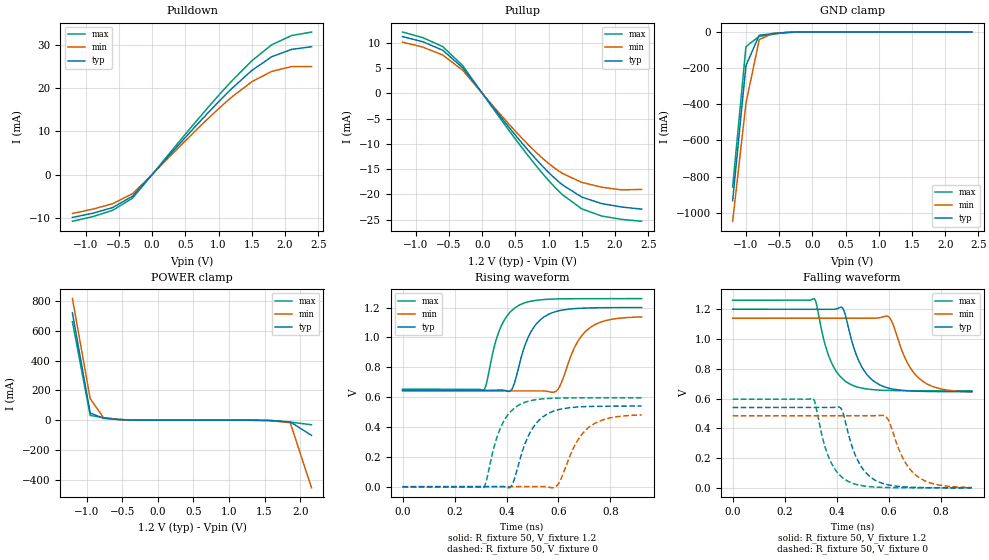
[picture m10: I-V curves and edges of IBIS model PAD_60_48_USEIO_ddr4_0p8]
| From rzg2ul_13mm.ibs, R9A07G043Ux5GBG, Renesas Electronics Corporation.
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[Model] PAD_60_48_USEIO_ddr4_0p8
Model_type I/O
Polarity   Non-Inverting
Vinl = 0.8670
Vinh = 1.0530
Vmeas= 0.960
| Capacitance   typ   min   max
C_comp   2.102e-12   2.013e-12   2.216e-12
[Model Spec]
| Subparameter   typ   min   max
Vmeas   0.960   0.912   1.008
Vinh   1.0530   1.0050   1.1010
Vinl   0.8670   0.8190   0.9150
| Variables   typ   min   max
[GND Clamp Reference]   0   0   0
[POWER Clamp Reference]   1.2   1.14   1.26
[Pulldown Reference]   0   0   0
[Pullup Reference]   1.2   1.14   1.26
[Temperature Range]   25   125   -40
[Voltage Range]   1.2   1.14   1.26
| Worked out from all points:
|   slope of the pulldown table from 0 to 0.18 V, typ, clamps not added: 57.7 ohm
|   slope of the pullup table from 0 to 0.18 V, typ, clamps not added: 59.2 ohm
|   GND clamp passes 1 mA (typ) near -0.30 V on its own axis
|   POWER clamp passes 1 mA (typ) near -0.38 V on its own axis
|   rising waveform, R_fixture 50, V_fixture 1.2: 20-80 % time 73.4ps typ, 82ps min, 66.5ps max; typ from 0.646 V to 1.2 V
|   rising waveform, R_fixture 50, V_fixture 0: 20-80 % time 78.4ps typ, 88.6ps min, 70.3ps max; typ from 0 V to 0.54 V
|   falling waveform, R_fixture 50, V_fixture 1.2: 20-80 % time 74.9ps typ, 84ps min, 68.9ps max; typ from 1.2 V to 0.646 V
|   falling waveform, R_fixture 50, V_fixture 0: 20-80 % time 73.8ps typ, 82.3ps min, 67.3ps max; typ from 0.54 V to 0 V
[GND Clamp]
| Voltage   I(typ)   I(min)   I(max)
-1.2V     -932.7mA   -1.047A    -857.4mA
-1V       -185.5mA   -394.3mA   -80.64mA
-800mV    -17.89mA   -41.9mA    -23.65mA
-600mV    -9.04mA    -7.411mA   -12.44mA
-400mV    -2.454mA   -2.378mA   -3.185mA
2.4V      0A         0A         0A
[POWER Clamp]
| Voltage   I(typ)   I(min)   I(max)
-1.2V     719.7mA    815.2mA    660.1mA
-950mV    48.1mA     144.6mA    32.07mA
-760mV    12.41mA    14.91mA    17.11mA
-360mV    527.4uA    791.2uA    575.5uA
1.26V     -115.5nA   -12.89uA   -796.6pA
1.56V     -1.53mA    -2.776mA   -549.4uA
1.86V     -11.39mA   -16.33mA   -12.44mA
2.16V     -101.5mA   -453.2mA   -30.39mA
[Pulldown]
| Voltage   I(typ)   I(min)   I(max)
-1.2V     -9.9mA     -9mA       -10.8mA
-895mV    -8.96mA    -8mA       -9.73mA
-595mV    -7.631mA   -6.738mA   -8.27mA
-295mV    -4.994mA   -4.407mA   -5.452mA
855mV     14.52mA    13.16mA    15.78mA
1.21V     20.07mA    18.08mA    21.85mA
1.5V      24.09mA    21.49mA    26.33mA
1.8V      27.28mA    23.9mA     30.05mA
2.1V      28.99mA    25mA       32.19mA
2.4V      29.6mA     25mA       33mA
[Pullup]
| Voltage   I(typ)   I(min)   I(max)
-1.2V     11.2mA     10.1mA     12.1mA
-895mV    10.18mA    9.12mA     11mA
-595mV    8.511mA    7.564mA    9.224mA
-295mV    5.039mA    4.554mA    5.475mA
300mV     -5.038mA   -4.584mA   -5.496mA
650mV     -10.64mA   -9.591mA   -11.66mA
955mV     -15.06mA   -13.39mA   -16.58mA
1.21V     -18.13mA   -15.86mA   -20.07mA
1.5V      -20.53mA   -17.62mA   -22.86mA
1.8V      -21.81mA   -18.57mA   -24.27mA
2.1V      -22.48mA   -19.1mA    -24.93mA
2.4V      -22.9mA    -19mA      -25.3mA
[Ramp]
dV/dt_r   0.3322/7.338e-11   0.2978/8.203e-11   0.3643/6.654e-11
dV/dt_f   0.3239/7.385e-11   0.2890/8.232e-11   0.3572/6.728e-11
R_load= 50
[Rising Waveform]
R_fixture = 50
V_fixture = 1.2
V_fixture_min = 1.14
V_fixture_max = 1.26
| Time   V(typ)   V(min)   V(max)
0s        646.4mV    641.1mV    652.8mV
312ps     646.4mV    641.1mV    646.5mV
364ps     646.7mV    641.1mV    1.006V
413ps     639.6mV    641.1mV    1.168V
493ps     1.035V     641.1mV    1.242V
583ps     1.17V      633.9mV    1.257V
608ps     1.181V     683.8mV    1.258V
666ps     1.194V     947.9mV    1.259V
708ps     1.197V     1.046V     1.26V
920ps     1.2V       1.137V     1.26V
[Rising Waveform]
R_fixture = 50
V_fixture = 0
V_fixture_min = 0
V_fixture_max = 0
| Time   V(typ)   V(min)   V(max)
0s        117.3nV    4.889uV    20.46nV
311ps     -237nV     4.778uV    -6.834mV
364ps     266.2uV    4.708uV    335.3mV
412ps     -6.394mV   12.92uV    496.4mV
491ps     364mV      -26.03uV   576mV
582ps     506.8mV    -5.953mV   592.9mV
606ps     518.9mV    38.49mV    594.2mV
670ps     533.7mV    299.7mV    595.5mV
716ps     537.5mV    396.4mV    595.9mV
920ps     540.2mV    480.9mV    596mV
[Falling Waveform]
R_fixture = 50
V_fixture = 1.2
V_fixture_min = 1.14
V_fixture_max = 1.26
| Time   V(typ)   V(min)   V(max)
0s        1.2V       1.14V      1.26V
314ps     1.2V       1.14V      1.27V
367ps     1.2V       1.14V      898.4mV
420ps     1.212V     1.14V      737.7mV
472ps     910.5mV    1.14V      681.3mV
501ps     799.7mV    1.14V      668.3mV
596ps     671.6mV    1.153V     654.3mV
672ps     652mV      840.5mV    652.5mV
716ps     648.4mV    737.4mV    652.2mV
920ps     645.9mV    644mV      652mV
[Falling Waveform]
R_fixture = 50
V_fixture = 0
V_fixture_min = 0
V_fixture_max = 0
| Time   V(typ)   V(min)   V(max)
0s        539.8mV    483.8mV    595.3mV
310ps     539.8mV    483.8mV    598.3mV
362ps     539.6mV    483.8mV    239.6mV
412ps     540.9mV    483.8mV    85.13mV
491ps     151.9mV    483.6mV    16.57mV
580ps     28.11mV    485.3mV    2.611mV
602ps     18.33mV    445.5mV    1.561mV
660ps     6.115mV    182.6mV    507.8uV
704ps     2.581mV    85.89mV    173.2uV
920ps     34.66uV    2.09mV     1.472uV
[Add Submodel]
| Submodel Name Mode
PAD_60_48_0p8_T Non-Driving
